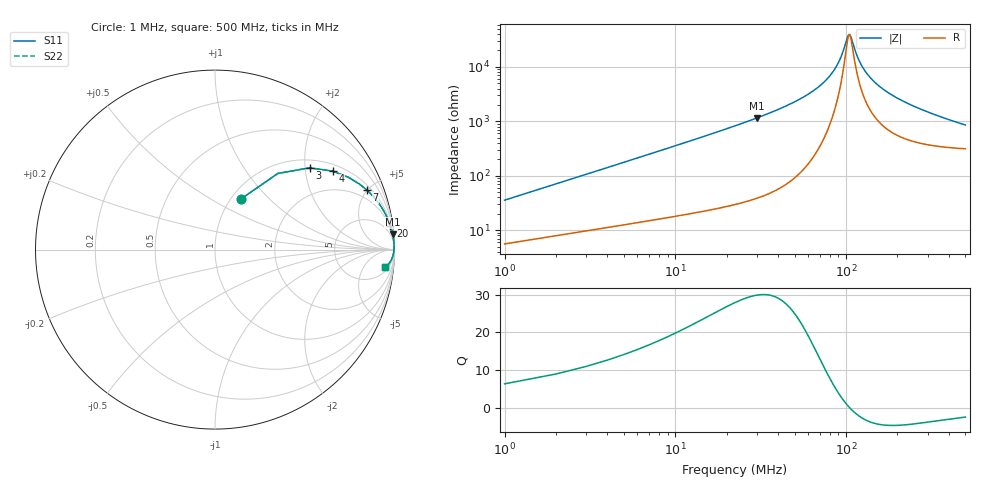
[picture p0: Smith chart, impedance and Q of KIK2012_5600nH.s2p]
!version-2
!date-01.2022
!Series
# MHz S RI R 50
!Freq ReS11 ImS11 ReS21 ImS21 ReS12 ImS12 ReS22 ImS22
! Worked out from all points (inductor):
!   500 points, 1 MHz to 500 MHz, reference 50 ohm
!   read as one part in series: L = 5.6 uH near 3 MHz
!   highest Q = 29.9 at 30 MHz (marker M1), where L = 6.1 uH
!   self-resonance near 104 MHz
!   S11 on the Smith chart (normalised r, x): 1 MHz: 1.11, +0.70; 3 MHz: 1.19, +2.11; 4 MHz: 1.22, +2.82; 7 MHz: 1.30, +4.95; 20 MHz: 2, +15; 500 MHz: 7, -16
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1  0.1476 0.284  0.8524 -0.284  0.8524 -0.284  0.1476 0.284
3  0.527 0.4556  0.473 -0.4556  0.473 -0.4556  0.527 0.4556
4  0.655 0.4373  0.345 -0.4373  0.345 -0.4373  0.655 0.4373
5  0.7428 0.403  0.2572 -0.403  0.2572 -0.403  0.7428 0.403
7  0.8456 0.3325  0.1544 -0.3325  0.1544 -0.3325  0.8456 0.3325
12  0.9393 0.2167  0.0607 -0.2167  0.0607 -0.2167  0.9393 0.2167
20  0.9769 0.1329  0.0231 -0.1329  0.0231 -0.1329  0.9769 0.1329
30  0.9897 0.0857  0.0103 -0.0857  0.0103 -0.0857  0.9897 0.0857
69  0.9978 0.0231  0.00224 -0.0231  0.00224 -0.0231  0.9978 0.0231
85  0.9979 0.0113  0.0021 -0.0113  0.0021 -0.0113  0.9979 0.0113
93  0.9978 0.00639  0.00221 -0.00639  0.00221 -0.00639  0.9978 0.00639
102  0.9976 0.00141  0.00244 -0.00141  0.00244 -0.00141  0.9976 0.00141
105  0.9975 -0.000151  0.00254 0.000151  0.00254 0.000151  0.9975 -0.000151
117  0.997 -0.00596  0.00302 0.00596  0.00302 0.00596  0.997 -0.00596
128  0.9964 -0.0108  0.00357 0.0108  0.00357 0.0108  0.9964 -0.0108
145  0.9954 -0.0176  0.00459 0.0176  0.00459 0.0176  0.9954 -0.0176
168  0.9937 -0.0259  0.00625 0.0259  0.00625 0.0259  0.9937 -0.0259
204  0.9906 -0.0374  0.00941 0.0374  0.00941 0.0374  0.9906 -0.0374
251  0.9856 -0.0506  0.0144 0.0506  0.0144 0.0506  0.9856 -0.0506
334  0.9749 -0.0702  0.0251 0.0702  0.0251 0.0702  0.9749 -0.0702
417  0.9623 -0.0862  0.0377 0.0862  0.0377 0.0862  0.9623 -0.0862
500  0.9487 -0.099  0.0513 0.099  0.0513 0.099  0.9487 -0.099
